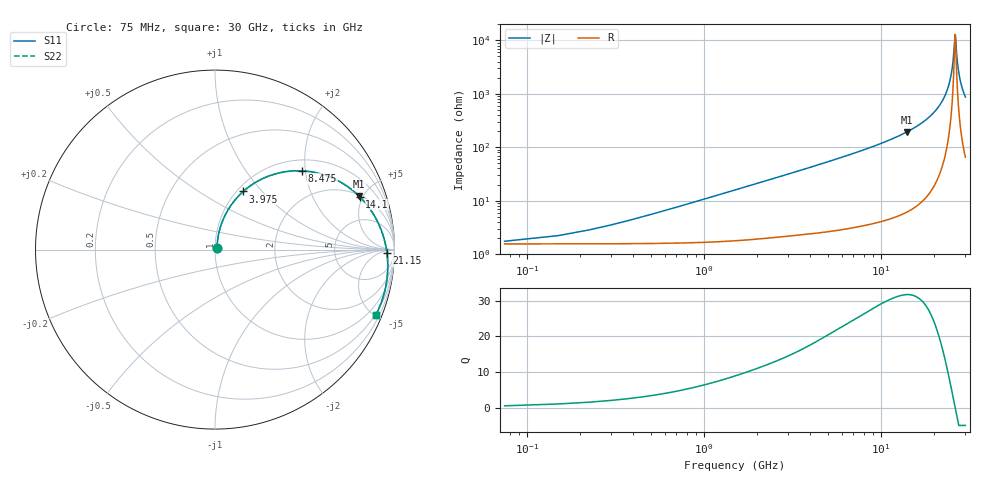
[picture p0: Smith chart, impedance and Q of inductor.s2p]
#  Hz  S  RI  R  50
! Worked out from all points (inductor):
!   400 points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, 75 MHz to 30 GHz, reference 50 ohm
!   read as one part in series: L = 1.67 nH near 450 MHz
!   highest Q = 31.7 at 14.03 GHz (marker M1), where L = 2.2 nH
!   self-resonance near 26.25 GHz
!   S11 on the Smith chart (normalised r, x): 75 MHz: 1.02, +0.01; 3.975 GHz: 1.07, +0.79; 8.475 GHz: 1.25, +1.92; 14.1 GHz: 2.11, +4.73; 21.15 GHz: 40, -17; 30 GHz: 0.44, -5.11
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7.5e7  0.0113 0.00713  0.9806 -0.00819  0.9806 -0.00819  0.0113 0.00712
2.25e8  0.0117 0.0214  0.98 -0.0245  0.98 -0.0245  0.0117 0.0214
4.5e8  0.0133 0.0427  0.9781 -0.049  0.9781 -0.049  0.0134 0.0426
1.125e9  0.0245 0.1054  0.9649 -0.1203  0.9649 -0.1203  0.0245 0.1054
2.25e9  0.0622 0.2028  0.9225 -0.2284  0.9225 -0.2284  0.0622 0.2026
3.975e9  0.1571 0.3239  0.8248 -0.3619  0.8248 -0.3619  0.1571 0.3237
5.1e9  0.235 0.3799  0.7468 -0.427  0.7468 -0.427  0.235 0.3796
8.475e9  0.4862 0.4388  0.4928 -0.5151  0.4928 -0.5151  0.4863 0.4382
1.005e10  0.5939 0.4209  0.384 -0.5107  0.384 -0.5107  0.594 0.4201
1.4025e10  0.8031 0.2981  0.1705 -0.4225  0.1705 -0.4225  0.8031 0.2969
1.41e10  0.8061 0.2951  0.1674 -0.4202  0.1674 -0.4202  0.8062 0.2939
1.5075e10  0.8425 0.2549  0.1299 -0.3885  0.1299 -0.3885  0.8425 0.2536
2.0025e10  0.9493 0.033  0.016 -0.21  0.016 -0.21  0.9489 0.0311
2.115e10  0.9583 -0.0175  0.00519 -0.1695  0.00519 -0.1695  0.9577 -0.0196
2.355e10  0.9622 -0.1214  -0.00322 -0.0868  -0.00322 -0.0868  0.9614 -0.1237
2.505e10  0.9559 -0.183  0.000226 -0.0386  0.000226 -0.0386  0.9548 -0.1854
2.565e10  0.9516 -0.2068  0.00322 -0.0202  0.00322 -0.0202  0.9505 -0.2093
2.625e10  0.9464 -0.2301  0.00707 -0.00234  0.00707 -0.00234  0.9452 -0.2327
2.7e10  0.9387 -0.2584  0.013 0.0192  0.013 0.0192  0.9374 -0.261
2.76e10  0.9317 -0.2803  0.0185 0.0358  0.0185 0.0358  0.9303 -0.283
2.8575e10  0.9189 -0.3147  0.029 0.0616  0.029 0.0616  0.9174 -0.3174
3e10  0.8974 -0.3626  0.0473 0.0965  0.0473 0.0965  0.8956 -0.3654
